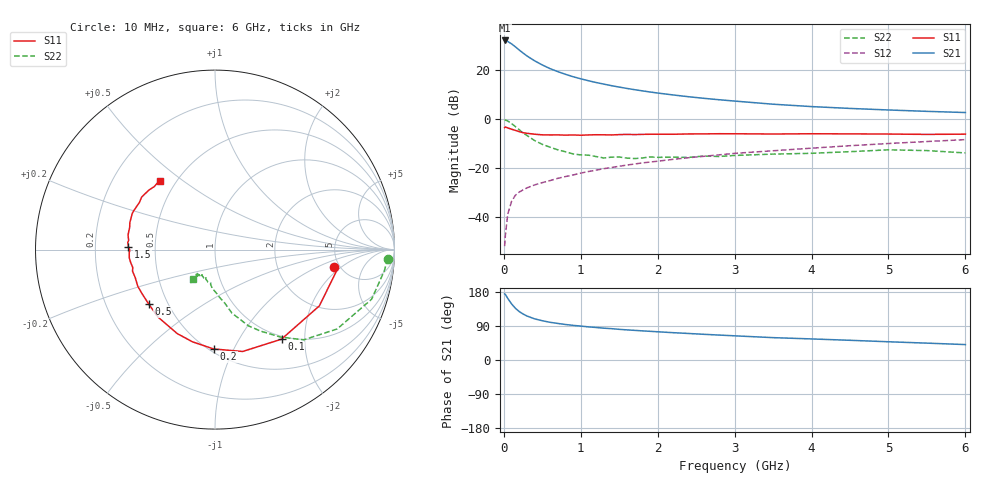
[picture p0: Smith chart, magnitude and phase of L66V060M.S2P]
!  INFINEON TECHNOLOGIES Small Signal Semiconductors
! BFR380L3 , Si-NPN RF-Transistor in TSLP-3-1
!  Vce=6 V,  Ic=60 mA
! Common Emitter S-Parameters:  07. March 2005
#  GHz  S  MA  R  50
! f  S11  S21  S12  S22
! GHz  Mag  Ang  Mag  Ang  Mag  Ang  Mag  Ang
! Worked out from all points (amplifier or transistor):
!   36 points, 10 MHz to 6 GHz, reference 50 ohm
!   highest |S21| = 32.0 dB at 10 MHz (marker M1)
!   |S21| within 3 dB of that: start of sweep to 165.9 MHz
!   unconditionally stable (mu >= 1): 1.573 GHz to 4.791 GHz
!   at 250 MHz: K = 0.47, MSG = 27.8 dB, |S12| = -28.8 dB
!   at 1.4 GHz: K = 0.99, MSG = 16.6 dB, |S12| = -19.7 dB
!   at 6 GHz: K = 0.97, MSG = 5.5 dB, |S12| = -8.4 dB
!   S11 on the Smith chart (normalised r, x): 10 MHz: 4.47, -1.54; 100 MHz: 0.95, -1.55; 200 MHz: 0.53, -0.84; 500 MHz: 0.39, -0.31; 1.5 GHz: 0.35, +0.02; 6 GHz: 0.41, +0.41
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0.01  0.668 -8.2  39.66 174.5  0.0026 76.6  0.9626 -3.0
0.02  0.6909 -9.0  39.33 173.0  0.0043 81.4  0.9514 -7.0
0.05  0.6607 -28.3  37.94 162.8  0.0115 75.5  0.9153 -17.6
0.1  0.6216 -53.4  33.85 148.2  0.0211 67.3  0.8116 -33.0
0.15  0.5882 -74.8  29.46 136.5  0.0282 60.9  0.7049 -45.5
0.2  0.5538 -90.7  25.33 127.8  0.0328 58.9  0.6084 -53.2
0.25  0.5289 -103.7  22.02 121.4  0.0362 55.0  0.5201 -60.8
0.3  0.5131 -114.2  19.24 116.1  0.0398 55.3  0.4641 -66.3
0.4  0.4921 -130.3  15.29 108.6  0.0458 55.4  0.3657 -75.1
0.5  0.4777 -140.8  12.59 103.6  0.0509 56.6  0.3057 -79.4
0.6  0.4749 -148.9  10.62 99.5  0.056 57.9  0.2681 -84.4
0.7  0.4763 -154.5  9.232 96.5  0.0622 60.0  0.2371 -89.2
0.8  0.4711 -160.4  8.139 93.7  0.0676 60.9  0.2163 -94.1
0.9  0.4748 -165.3  7.26 91.4  0.0729 62.2  0.1956 -97.2
1.1  0.4754 -171.4  6.013 87.4  0.0858 63.9  0.1845 -102.3
1.5  0.4831 178.0  4.467 80.9  0.1097 66.1  0.1694 -111.8
1.8  0.4879 172.0  3.746 76.9  0.1283 66.5  0.1614 -116.8
2.2  0.491 165.6  3.093 72.1  0.1517 66.7  0.168 -120.1
3.5  0.4964 147.9  2.004 59.0  0.2266 64.6  0.1939 -126.6
4.5  0.4992 141.9  1.645 52.0  0.2872 63.2  0.2172 -126.6
5.5  0.4876 134.0  1.434 44.5  0.3492 59.6  0.2284 -126.4
6  0.4933 128.8  1.357 40.7  0.3818 57.6  0.2046 -127.2
